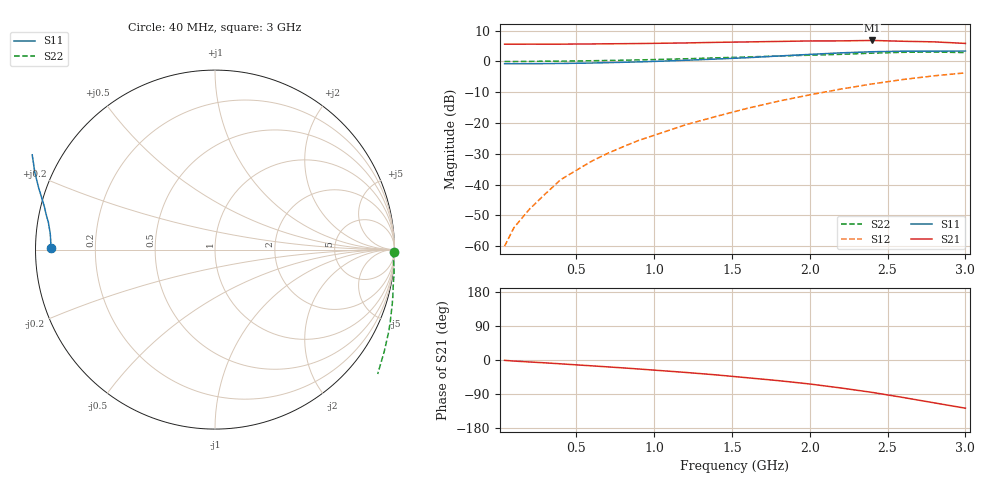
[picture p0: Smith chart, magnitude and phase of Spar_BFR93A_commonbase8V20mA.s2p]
! Filename:  BFR93ACG.S2P  Version:  2.0
! NXP part #: BFR93A  Date: Jul 1990
! Bias condition: Vce=8V, Ic=20mA
! COMMON BASE
#  MHz  S  MA  R  50
! Freq  S11  S21  S12  S22
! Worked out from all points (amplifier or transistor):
!   21 points, 40 MHz to 3 GHz, reference 50 ohm
!   highest |S21| = 6.8 dB at 2.4 GHz (marker M1)
!   |S21| within 3 dB of that: start of sweep to end of sweep
!   unconditionally stable (mu >= 1): start of sweep to 45.33 MHz
!   at 300 MHz: K = -0.62, MSG = 24.3 dB, |S12| = -43.1 dB
!   at 1 GHz: K = -0.93, MSG = 14.9 dB, |S12| = -24.0 dB
!   at 3 GHz: K = -0.83, MSG = 4.8 dB, |S12| = -3.7 dB
40  0.916 179.3  1.901 -0.9  0.001 38.6  0.995 -0.8
100  0.915 178.2  1.9 -2.8  0.002 84.7  0.994 -2.5
200  0.917 176.8  1.903 -5.2  0.004 109.2  0.999 -4.7
300  0.92 175.3  1.901 -7.5  0.007 122.5  1.006 -7.1
400  0.925 173.8  1.902 -10.1  0.012 131.8  1.009 -9.6
500  0.932 172.4  1.912 -12.8  0.017 137.2  1.015 -12.1
600  0.94 170.8  1.918 -15.4  0.024 140.0  1.024 -14.6
700  0.953 169.2  1.929 -18.1  0.032 141.6  1.034 -17.3
800  0.966 167.6  1.936 -20.8  0.041 143.1  1.044 -19.9
900  0.981 165.8  1.947 -23.7  0.052 144.3  1.056 -22.4
1000  0.998 164.2  1.962 -26.7  0.063 143.9  1.07 -25.2
1200  1.041 160.7  1.99 -32.7  0.093 143.5  1.101 -31.1
1400  1.091 156.9  2.036 -39.3  0.128 141.0  1.141 -37.4
1600  1.147 152.6  2.068 -46.9  0.173 138.5  1.181 -44.1
1800  1.222 147.6  2.107 -54.5  0.226 134.3  1.22 -51.6
2000  1.298 142.3  2.145 -63.3  0.286 129.2  1.26 -60.3
2200  1.375 136.6  2.15 -73.8  0.355 123.3  1.301 -70.6
2400  1.433 129.6  2.185 -85.4  0.43 115.9  1.359 -81.8
2600  1.463 121.5  2.12 -98.9  0.508 108.0  1.403 -93.0
2800  1.467 111.8  2.072 -113.1  0.583 98.9  1.418 -104.7
3000  1.47 102.0  1.957 -127.2  0.651 90.9  1.388 -116.2
